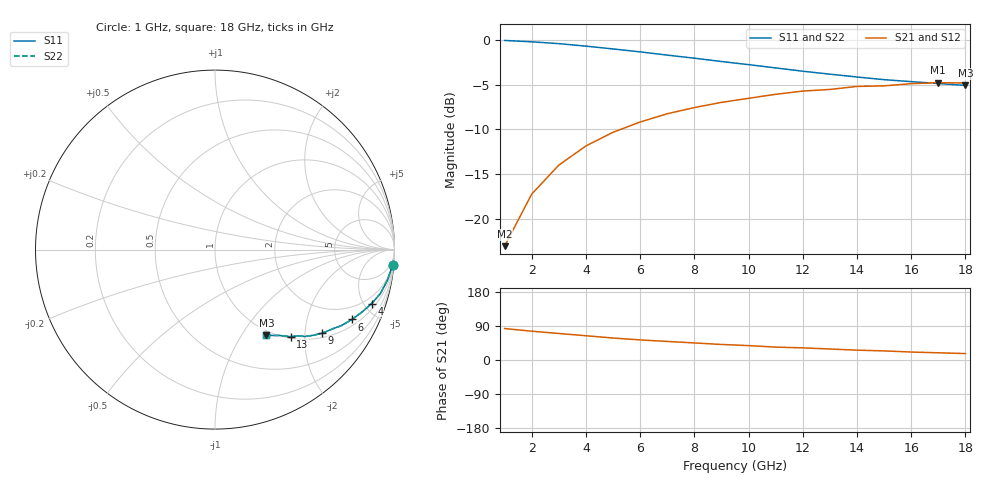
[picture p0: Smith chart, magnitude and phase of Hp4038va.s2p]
!HPND-4038 beam lead PIN diode
!Series configuration S-parameters Vr= 0 V.  Last updated 10/3/97
# mhz s ma r 50
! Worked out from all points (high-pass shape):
!   18 points, 1 GHz to 18 GHz, reference 50 ohm
!   highest |S21| = -4.79 dB at 17 GHz (marker M1); lowest = -23.1 dB at 1 GHz (marker M2)
!   |S21| within 3 dB of the highest: 7.689 GHz to end of sweep
!   lowest |S11| = -5.1 dB at 18 GHz (marker M3), VSWR 3.50, Z = 46.9 - j64.7 ohm
!   |S11| at or under -10 dB: nowhere
!   |S22| runs from -5.1 to -0.1 dB; largest |S21 - S12| = 0
!   S11 on the Smith chart (normalised r, x): 1 GHz: 2, -23; 4 GHz: 1.39, -5.64; 6 GHz: 1.28, -3.75; 9 GHz: 1.12, -2.45; 13 GHz: 1.03, -1.70; 18 GHz: 0.94, -1.29
1000  0.993 -5.0  0.07 83.0  0.07 83.0  0.993 -5.0
2000  0.976 -10.0  0.137 76.0  0.137 76.0  0.976 -10.0
3000  0.953 -15.0  0.199 70.0  0.199 70.0  0.953 -15.0
4000  0.923 -19.0  0.255 64.0  0.255 64.0  0.923 -19.0
5000  0.89 -23.0  0.304 58.0  0.304 58.0  0.89 -23.0
6000  0.857 -27.0  0.347 53.0  0.347 53.0  0.857 -27.0
7000  0.822 -31.0  0.386 49.0  0.386 49.0  0.822 -31.0
8000  0.79 -34.0  0.418 45.0  0.418 45.0  0.79 -34.0
9000  0.757 -38.0  0.447 41.0  0.447 41.0  0.757 -38.0
10000  0.727 -41.0  0.471 38.0  0.471 38.0  0.727 -41.0
11000  0.697 -44.0  0.496 34.0  0.496 34.0  0.697 -44.0
12000  0.668 -46.0  0.517 32.0  0.517 32.0  0.668 -46.0
13000  0.643 -49.0  0.528 29.0  0.528 29.0  0.643 -49.0
14000  0.62 -51.0  0.549 26.0  0.549 26.0  0.62 -51.0
15000  0.599 -53.0  0.553 24.0  0.553 24.0  0.599 -53.0
16000  0.584 -55.0  0.569 21.0  0.569 21.0  0.584 -55.0
17000  0.57 -57.0  0.576 19.0  0.576 19.0  0.57 -57.0
18000  0.556 -59.0  0.574 17.0  0.574 17.0  0.556 -59.0
